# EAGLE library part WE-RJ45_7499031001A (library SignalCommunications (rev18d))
WE-RJ45 LAN Transformer Order Code 7499031001A Design THT xBase-T 10/100 Base-T Ports 1x4 Application Standard Tab Position DOWN LED (Left-Right) NO EMI Fingers No Details see: http://katalog.we-online.de/en/pbs/WE-LAN-RJ45 Created by Yingchun Shan 2016 (C) Wurth Elektronik
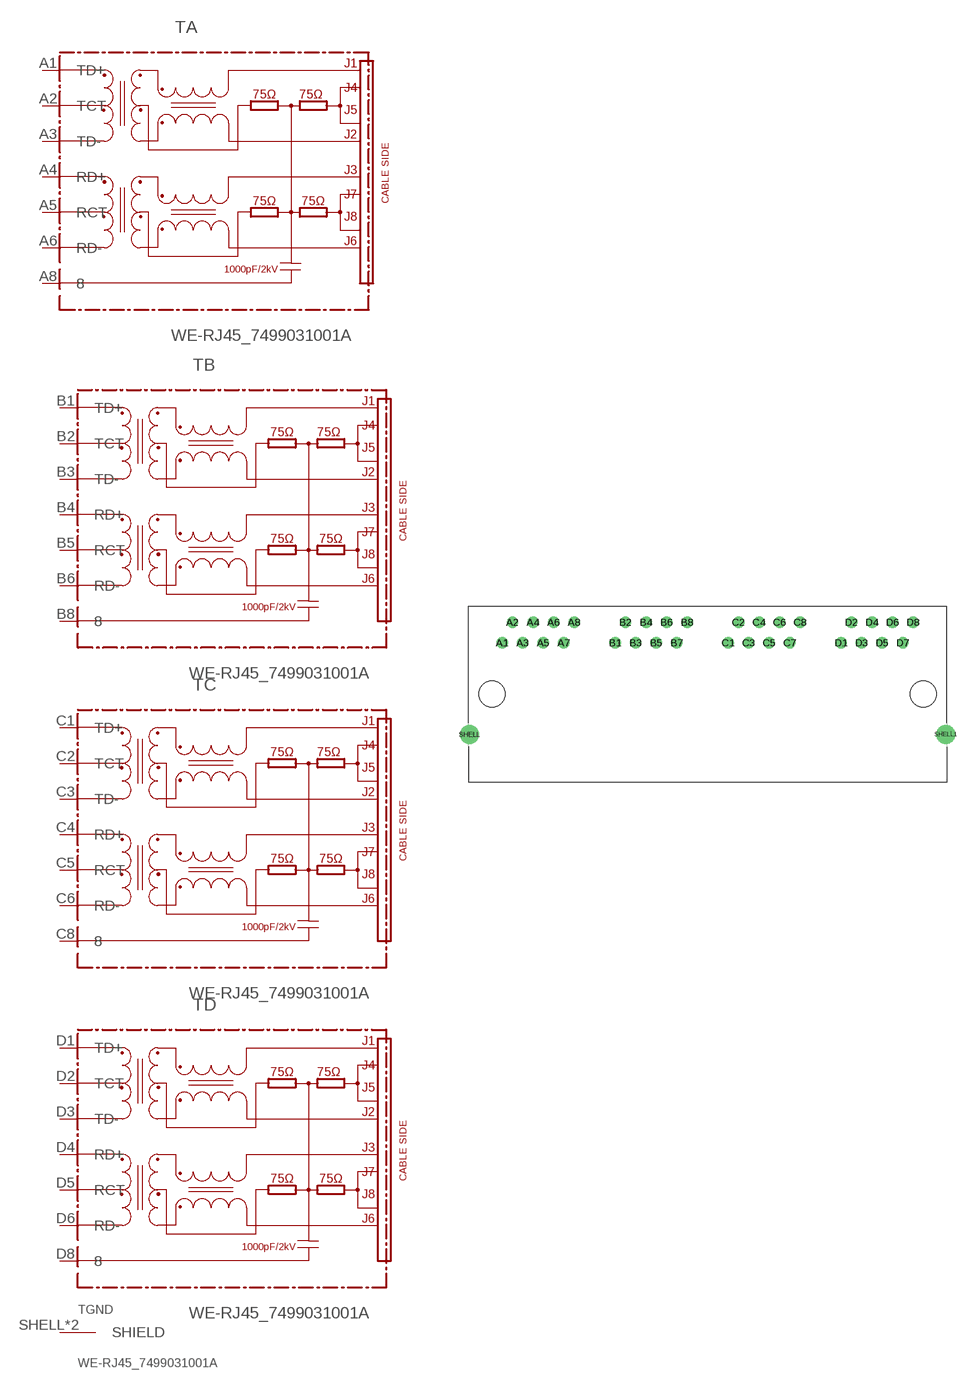
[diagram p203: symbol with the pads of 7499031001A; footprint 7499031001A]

Designator prefix T; gates A=7499021002A B=7499021002A C=7499021002A D=7499021002A GND=SHIELD

## WE-RJ45_7499031001A  [7499031001A]
A1  A:TD+
A2  A:TCT
A3  A:TD-
A4  A:RD+
A5  A:RCT
A6  A:RD-
A8  A:8
B1  B:TD+
B2  B:TCT
B3  B:TD-
B4  B:RD+
B5  B:RCT
B6  B:RD-
B8  B:8
C1  C:TD+
C2  C:TCT
C3  C:TD-
C4  C:RD+
C5  C:RCT
C6  C:RD-
C8  C:8
D1  D:TD+
D2  D:TCT
D3  D:TD-
D4  D:RD+
D5  D:RCT
D6  D:RD-
D8  D:8
SHELL  GND:SHIELD  pas
SHELL1  GND:SHIELD  pas

## Footprint 7499031001A (pad centres in mm)
drill 0.9: A1 -25.4,6.35; A2 -24.13,8.89; A3 -22.86,6.35; A4 -21.59,8.89; A5 -20.32,6.35; A6 -19.05,8.89; A7 -17.78,6.35; A8 -16.51,8.89; B1 -11.43,6.35; B2 -10.16,8.89; B3 -8.89,6.35; B4 -7.62,8.89; B5 -6.35,6.35; B6 -5.08,8.89; B7 -3.81,6.35; B8 -2.54,8.89; C1 2.54,6.35; C2 3.81,8.89; C3 5.08,6.35; C4 6.35,8.89; C5 7.62,6.35; C6 8.89,8.89; C7 10.16,6.35; C8 11.43,8.89; D1 16.51,6.35; D2 17.78,8.89; D3 19.05,6.35; D4 20.32,8.89; D5 21.59,6.35; D6 22.86,8.89; D7 24.13,6.35; D8 25.4,8.89
drill 1.57: SHELL -29.455,-5; SHELL1 29.455,-5
hole 3.2 at -26.67,0
hole 3.2 at 26.67,0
